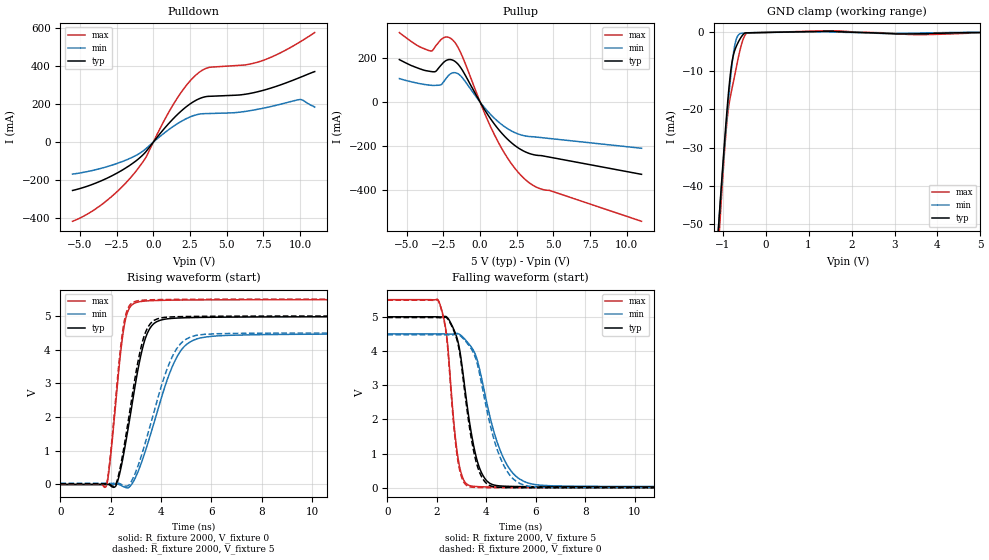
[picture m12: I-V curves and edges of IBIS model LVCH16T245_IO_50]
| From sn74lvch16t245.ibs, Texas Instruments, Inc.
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[Model]   LVCH16T245_IO_50
Model_type  I/O
Vinl=1.35
Vinh=3.85
Enable   Active-Low
Vref =   0
Rref =   2000
Cref =   15p
Vmeas =   2.5
| variable   typ   min   max
C_comp   5.69pF   4.67pF   7.26pF
| C_pullup   14.81pF   6.00pF   28.04pF
| C_pulldown   8.87pF   6.27pF   14.48pF
| C_tri-state   5.69pF   4.67pF   7.26pF
[Temperature Range]   40   100   -40
| Ambient temperature   25   85   -40
[Voltage range]   5   4.5   5.5
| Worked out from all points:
|   slope of the pulldown table from 0 to 0.75 V, typ, clamps not added: 10.5 ohm
|   slope of the pullup table from 0 to 0.75 V, typ, clamps not added: 9.47 ohm
|   GND clamp passes 1 mA (typ) near -0.56 V on its own axis
|   rising waveform, R_fixture 2000, V_fixture 0: 20-80 % time 708ps typ, 1.16ns min, 440ps max; typ from 0 V to 4.98 V
|   falling waveform, R_fixture 2000, V_fixture 5: 20-80 % time 622ps typ, 977ps min, 403ps max; typ from 5 V to 0.025 V
|   rising waveform, R_fixture 2000, V_fixture 5: 20-80 % time 679ps typ, 1.09ns min, 428ps max; typ from 0.025 V to 5 V
|   falling waveform, R_fixture 2000, V_fixture 0: 20-80 % time 598ps typ, 906ps min, 393ps max; typ from 4.98 V to 0 V
[GND Clamp]
| LVCH16T245_IO_50
|   Voltage   I(typ)   I(min)   I(max)
-5.5V     -898.4mA   -832.8mA   -1.017A
-1.115V   -53.75mA   -53.26mA   -59.03mA
-1.08V    -47.95mA   -47.91mA   -52.5mA
-1.05V    -43.07mA   -43.39mA   -47.02mA
-960mV    -28.99mA   -30.28mA   -31.6mA
-910mV    -21.74mA   -23.39mA   -24.41mA
-870mV    -16.44mA   -18.19mA   -20.15mA
-810mV    -9.91mA    -11.12mA   -16.1mA
-710mV    -4.401mA   -2.896mA   -10.66mA
-595mV    -1.669mA   -322.7uA   -4.527mA
-430mV    -101uA     -95.24uA   -160uA
5V        47.91pA    410.1nA    -73.17uA
[Pulldown]
| LVCH16T245_IO_50
|   Voltage   I(typ)   I(min)   I(max)
-5.5V     -253.9mA   -167.8mA   -415.9mA
-3.43V    -199.2mA   -134.9mA   -323mA
-1.42V    -112.1mA   -79.11mA   -175.4mA
-515mV    -51.25mA   -34.88mA   -81.44mA
675mV     64.66mA    43.62mA    103.8mA
1.605V    142.3mA    95.28mA    227.8mA
2.375V    193.6mA    128.1mA    310mA
3.085V    226.9mA    146.6mA    364.6mA
3.83V     241.1mA    150.7mA    393.4mA
7.4V      270.6mA    177.1mA    427.6mA
10.03V    341.2mA    224.3mA    528.3mA
11V       371.1mA    184.2mA    576.2mA
[Pullup]
| LVCH16T245_IO_50
|   Voltage   I(typ)   I(min)   I(max)
-5.5V     192.6mA    106.5mA    315.1mA
-3.39V    139mA      76.44mA    232.1mA
-3.02V    139.4mA    75.83mA    254.6mA
-2.445V   182.3mA    95.48mA    292.9mA
-1.78V    187.3mA    133.5mA    275.4mA
-1.265V   150.4mA    114.7mA    215.4mA
270mV     -30.29mA   -22.56mA   -44.29mA
1.205V    -119.5mA   -87.17mA   -177.6mA
2.245V    -190.4mA   -134.4mA   -289.3mA
3.285V    -231.3mA   -155.7mA   -362.5mA
4.095V    -242.4mA   -160.5mA   -392.8mA
11V       -327.5mA   -209.3mA   -540.4mA
[Ramp]
| LVCH16T245_IO_50
| variable   typ   min   max
dV/dt_r   3.04/7.20E-10   2.74/1.19E-09   3.34/4.46E-10
dV/dt_f   2.99/6.26E-10   2.69/9.84E-10   3.30/4.07E-10
R_load = 2000
[Rising Waveform]
| LVCH16T245_IO_50
R_fixture =   2000
C_fixture =   0
L_fixture =   0
V_fixture =   0
V_fixture_min = 0
V_fixture_max = 0
|   Time   V(typ)   V(min)   V(max)
0s        493.7pV    5.719nV    1.84nV
1.825ns   3.501mV    -45.7uV    -38.66mV
2.21ns    -31.37mV   7.505mV    2.513V
2.53ns    970.8mV    -71.46mV   4.683V
3.08ns    3.402V     373.5mV    5.413V
3.38ns    4.344V     1.003V     5.444V
3.72ns    4.778V     1.83V      5.457V
4.645ns   4.938V     3.804V     5.472V
5.57ns    4.957V     4.35V      5.477V
29.99ns   4.978V     4.473V     5.483V
[Falling Waveform]
| LVCH16T245_IO_50
R_fixture =   2000
C_fixture =   0
L_fixture =   0
V_fixture =   5
V_fixture_min = 4.5
V_fixture_max = 5.5
|   Time   V(typ)   V(min)   V(max)
0s        5V         4.5V       5.5V
2.085ns   4.997V     4.5V       5.449V
2.395ns   4.997V     4.497V     4.48V
2.875ns   4.212V     4.503V     794.7mV
3.35ns    1.798V     4.16V      62.07mV
3.665ns   712.7mV    3.656V     35.86mV
4.035ns   193.3mV    2.441V     28.43mV
4.82ns    45.88mV    694.1mV    23.17mV
5.845ns   34.41mV    112.1mV    20.98mV
29.99ns   24.87mV    33.38mV    16.99mV
[Rising Waveform]
| LVCH16T245_IO_50
R_fixture =   2000
C_fixture =   0
L_fixture =   0
V_fixture =   5
V_fixture_min = 4.5
V_fixture_max = 5.5
|   Time   V(typ)   V(min)   V(max)
0s        24.78mV    32.91mV    16.98mV
1.815ns   27.56mV    32.88mV    -27.56mV
2.195ns   -383.6uV   39.42mV    2.544V
2.505ns   1.021V     -27.95mV   4.707V
3.03ns    3.436V     445.5mV    5.444V
3.33ns    4.409V     1.13V      5.471V
3.655ns   4.834V     1.979V     5.481V
4.515ns   4.975V     3.894V     5.491V
5.395ns   4.987V     4.425V     5.495V
29.99ns   5V         4.5V       5.5V
[Falling Waveform]
| LVCH16T245_IO_50
R_fixture =   2000
C_fixture =   0
L_fixture =   0
V_fixture =   0
V_fixture_min = 0
V_fixture_max = 0
|   Time   V(typ)   V(min)   V(max)
0s        4.979V     4.474V     5.484V
2.085ns   4.976V     4.475V     5.431V
2.39ns    4.977V     4.471V     4.457V
2.86ns    4.194V     4.48V      758.3mV
3.32ns    1.777V     4.141V     34.26mV
3.62ns    682.7mV    3.669V     11.38mV
3.97ns    157.2mV    2.463V     6.105mV
4.71ns    10.38mV    650.9mV    3.014mV
5.655ns   3.623mV    54.98mV    1.966mV
29.99ns   76.68uV    274.5uV    10.32uV
